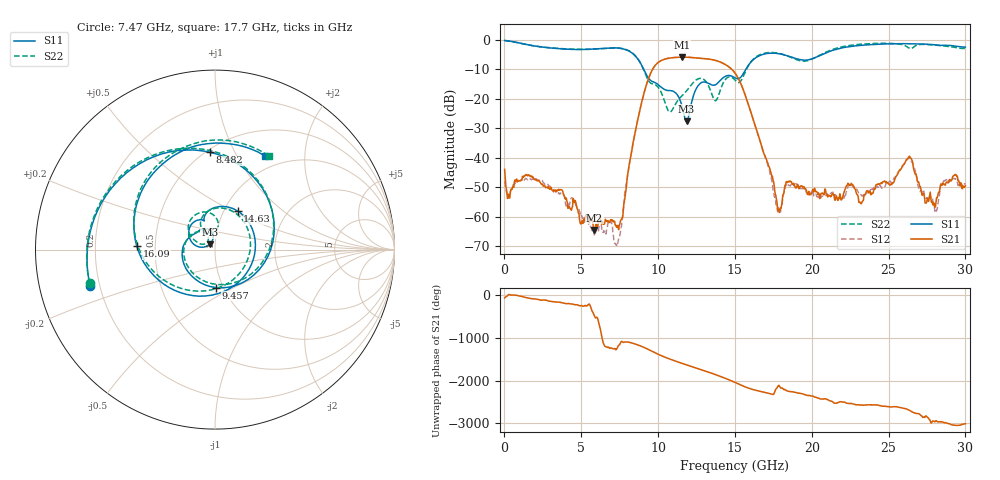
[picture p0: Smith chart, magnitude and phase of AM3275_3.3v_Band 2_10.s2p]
!Keysight Technologies,N5245B,MY58422270,A.16.20.02
!Date: Thursday, March 27, 2025 01:53:20
!Correction: S11(C  2-Port  )
!S21(C  2-Port  )
!S12(C  2-Port  )
!S22(C  2-Port  )
!S2P File: Measurements: S11, S21, S12, S22:
# Hz S  dB  R 50
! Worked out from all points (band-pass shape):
!   801 points, 10 MHz to 30 GHz, reference 50 ohm
!   highest |S21| = -5.86 dB at 11.56 GHz (marker M1); lowest = -64.5 dB at 5.858 GHz (marker M2)
!   |S21| within 3 dB of the highest: 9.782 GHz to 14.53 GHz (4.747 GHz wide, 39.1 % of centre)
!   lowest |S11| = -27.5 dB at 11.86 GHz (marker M3), VSWR 1.09, Z = 47.1 + j2.87 ohm
!   |S11| at or under -10 dB: 9.067 GHz to 15.71 GHz (6.64 GHz wide, 53.6 % of centre)
!   |S22| runs from -24.4 to -0.2 dB; largest |S21 - S12| = 0.01
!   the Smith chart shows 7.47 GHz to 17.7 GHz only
!   S11 on the Smith chart (normalised r, x): 7.47 GHz: 0.16, -0.14; 8.482 GHz: 0.52, +0.80; 9.457 GHz: 0.92, -0.41; 14.63 GHz: 1.16, +0.53; 16.09 GHz: 0.39, +0.02; 17.7 GHz: 0.82, +1.32
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1e7  -0.20 -5.2  -43.90 -59.3  -47.97 110.9  -0.20 -6.2
8.722125e8  -0.93 -85.6  -47.96 -2.6  -47.95 -9.6  -0.96 -85.6
2.034325e9  -2.12 -171.7  -47.25 -83.2  -47.08 -84.6  -2.13 -172.0
3.533825e9  -2.98 103.4  -50.62 -157.7  -52.11 -164.1  -2.91 102.7
5.033325e9  -3.27 18.7  -61.39 121.2  -59.59 112.0  -3.22 17.5
5.85805e9  -3.09 -35.3  -64.46 -127.4  -66.49 -79.8  -3.12 -36.8
7.470012e9  -2.80 -163.7  -62.80 -85.2  -67.10 62.4  -2.82 -164.9
8.482175e9  -5.29 93.2  -31.93 -59.3  -32.01 -59.8  -5.15 92.8
9.45685e9  -13.50 -88.7  -12.01 153.5  -12.00 153.3  -14.39 -94.7
1.001916e10  -15.25 168.2  -7.60 54.3  -7.60 54.0  -16.16 148.5
1.155615e10  -22.56 97.6  -5.86 -157.2  -5.86 -157.3  -18.93 156.7
1.185605e10  -27.54 133.6  -5.88 166.4  -5.87 166.4  -17.26 153.8
1.32056e10  -14.55 117.5  -6.46 6.1  -6.44 5.9  -14.82 89.1
1.463012e10  -12.07 59.5  -9.24 174.1  -9.24 174.1  -12.57 77.7
1.5005e10  -12.89 7.1  -11.24 115.2  -11.24 115.2  -13.63 21.5
1.609214e10  -7.20 177.5  -25.35 -43.1  -25.43 -43.3  -7.14 174.3
1.77041e10  -4.56 61.8  -54.11 -29.6  -56.08 171.1  -4.41 59.8
2.002832e10  -6.40 -123.6  -51.29 157.8  -51.36 153.0  -6.47 -130.9
2.25025e10  -2.25 104.9  -49.38 -23.5  -49.05 -14.8  -1.87 103.1
2.501416e10  -1.35 38.9  -48.71 -94.2  -48.15 -91.0  -1.17 35.7
2.748834e10  -1.47 -22.7  -54.81 31.5  -53.56 150.8  -1.58 -22.1
3e10  -2.46 -109.9  -49.36 -135.8  -48.90 -146.1  -2.90 -111.1
